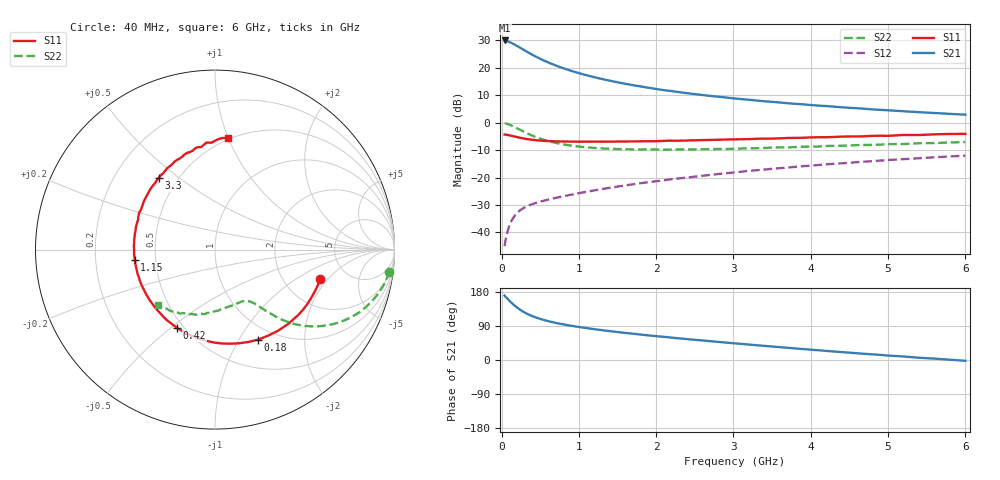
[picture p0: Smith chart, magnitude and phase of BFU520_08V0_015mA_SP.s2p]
! Filename:  P:\Prog\Test\Noise\ATS_data\Testdata_Net\03 Spar\BFU520_APG2013_37_A05_08p0V_015mA_SP_CM01_D.s2p
! Date/Time: Fri 26/Apr/2013 13:00:10
! BFU520_APG2013_37_A05_08p0V_1to20mA_SP_CM01_Bias7_R.s2p
! MDIF S-parameter v. bias file
! BFU520_APG2013_37_A05_08p0V_1to20mA_SP_CM01
! Date/time Tue Apr 23 17:06:44 2013
! VAR V_out= 8.0000
! VAR I_out= 14.9900
! VAR V_in= 0.8258
! VAR I_in= 0.1661
! Device data file deembeded for feedlines and parallel
! Original file: \03 Spar\BFU520_APG2013_37_A05_08p0V_015mA_SP_CM01_R.s2p
! Feed-files: PR047V01_250413_Feed1.s2p, PR047V01_250413_Feed2.s2p
! Parallel-file: PR047V01_250413_Par.s2p
# MHz S MA R 50
!  Freq-MHz  S11-mag  S11-arg  S21-mag  S21-arg  S12-mag  S12-arg  S22-mag  S22-arg
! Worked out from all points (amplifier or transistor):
!   98 points, 40 MHz to 6 GHz, reference 50 ohm
!   highest |S21| = 30.0 dB at 40 MHz (marker M1)
!   |S21| within 3 dB of that: start of sweep to 261.6 MHz
!   unconditionally stable (mu >= 1): 1.56 GHz to 3.574 GHz
!   at 300 MHz: K = 0.39, MSG = 28.6 dB, |S12| = -30.9 dB
!   at 1.6 GHz: K = 1.01, MAG = 18.0 dB, |S12| = -22.9 dB
!   at 6 GHz: K = 0.85, MSG = 7.5 dB, |S12| = -12.0 dB
!   S11 on the Smith chart (normalised r, x): 40 MHz: 3.19, -1.66; 180 MHz: 0.83, -1.21; 420 MHz: 0.46, -0.52; 1.15 GHz: 0.38, -0.05; 3.3 GHz: 0.39, +0.42; 6 GHz: 0.49, +1.00
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40  0.6092 -15.6  31.64 170.0  0.005597 83.0  0.9765 -7.2
50  0.6057 -19.6  31.59 167.1  0.006885 81.6  0.9726 -9.0
90  0.5937 -34.5  30 158.9  0.01187 75.7  0.9353 -16.1
120  0.5815 -45.3  28.9 152.7  0.01525 71.6  0.8997 -20.9
140  0.5726 -52.0  27.99 148.8  0.01728 69.1  0.8741 -23.8
180  0.556 -64.6  26.08 141.9  0.0209 64.8  0.8207 -28.8
220  0.5385 -75.9  24.28 135.5  0.02386 61.5  0.7677 -33.0
300  0.5112 -94.8  20.83 125.3  0.02851 56.8  0.673 -39.3
360  0.4964 -106.5  18.61 119.2  0.03129 54.6  0.6146 -42.7
420  0.4844 -116.0  16.72 114.2  0.03359 53.4  0.5647 -45.1
550  0.4662 -132.9  13.6 105.4  0.03776 52.4  0.4846 -48.5
650  0.4601 -142.4  11.83 100.3  0.04104 52.4  0.4452 -50.3
800  0.4546 -153.7  9.848 94.0  0.04555 53.2  0.4025 -52.1
1050  0.4503 -168.4  7.674 85.6  0.05335 54.8  0.3615 -54.8
1150  0.4503 -172.9  7.041 82.7  0.05657 55.4  0.351 -55.8
1600  0.4537 169.9  5.129 71.5  0.07169 56.9  0.328 -61.5
2050  0.4635 157.6  4.02 62.0  0.08712 57.3  0.3232 -68.4
3100  0.4989 132.2  2.696 42.5  0.1276 54.9  0.3383 -86.0
3300  0.5087 128.1  2.538 39.0  0.1359 54.0  0.3426 -89.4
4100  0.5429 112.8  2.05 25.7  0.169 49.5  0.3681 -103.4
5200  0.598 94.6  1.618 9.3  0.2166 41.7  0.4082 -122.4
6000  0.6249 83.3  1.402 -2.1  0.2508 35.0  0.4454 -135.9
